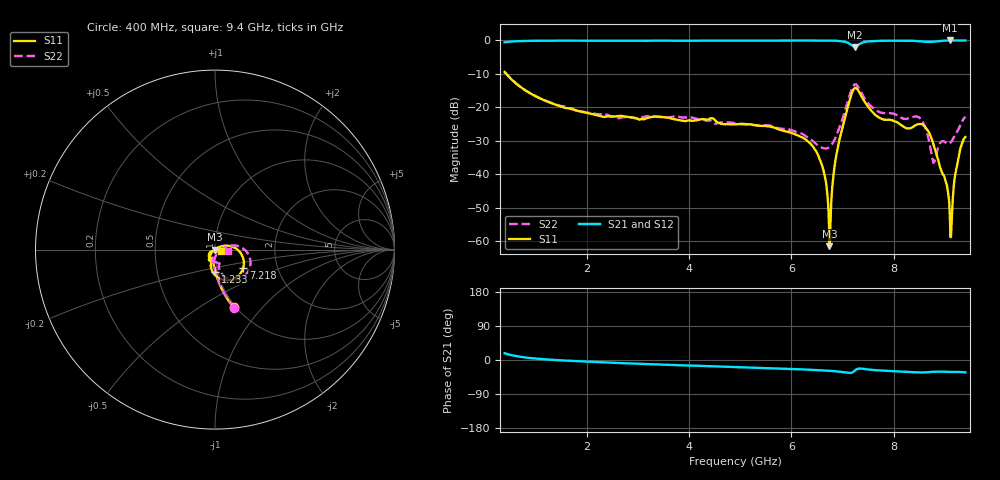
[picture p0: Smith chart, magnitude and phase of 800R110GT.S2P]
!  American Technical Ceramics  Date:  10/25/10
!  One Norden Lane
!  Huntington Station,  NY.  11746-2102
!  Tel:  (631) 622-4700  Fax:  (631) 622-4748
!  Part Number  800R110GT  Mounting Orientation: Vertical
!  Description: Ultra Low ESR Microwave Capacitor
!  Application: Coupling, Bypass, Tuning, DC Block, Filters, Matching
# GHZ S DB R 50
! Freq  |S11|  S11 Ph  |S21|  S21 Ph  |S12|  S12 Ph  |S22|  S22 Ph
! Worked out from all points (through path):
!   801 points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, 400 MHz to 9.4 GHz, reference 50 ohm
!   highest |S21| = 0.00 dB at 9.096 GHz (marker M1); lowest = -1.9 dB at 7.24 GHz (marker M2)
!   group delay of S21, straight-line fit = 12.8 ps
!   lowest |S11| = -61.5 dB at 6.745 GHz (marker M3), VSWR 1.00, Z = 49.9 + j0.0208 ohm
!   |S11| at or under -10 dB: 432.9 MHz to end of sweep
!   |S22| runs from -36.6 to -9.4 dB; largest |S21 - S12| = 0.0024
!   S11 on the Smith chart (normalised r, x): 400 MHz: 0.98, -0.71; 1.233 GHz: 0.97, -0.24; 7.218 GHz: 1.34, -0.28; 9.4 GHz: 1.07, -0.01
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0.4  -9.40 -72.1  -0.53 18.0  -0.53 18.0  -9.37 -71.9
1.233  -18.26 -89.0  -0.07 1.4  -0.07 1.3  -18.20 -88.2
1.908  -21.35 -94.8  -0.05 -3.8  -0.04 -3.8  -21.20 -93.0
3.404  -22.74 -104.4  -0.04 -11.6  -0.03 -11.7  -22.85 -98.3
4.9  -25.07 -116.7  -0.04 -18.6  -0.04 -18.7  -24.72 -100.8
6.408  -31.44 -137.2  -0.01 -26.0  -0.01 -26.0  -29.91 -79.8
6.633  -39.12 -141.8  -0.04 -27.6  -0.04 -27.7  -32.24 -49.6
6.745  -61.50 165.7  -0.05 -28.5  -0.06 -28.6  -31.84 -25.2
6.779  -48.62 47.8  -0.06 -28.9  -0.07 -28.9  -31.29 -17.3
6.824  -40.27 38.4  -0.08 -29.3  -0.09 -29.4  -30.27 -7.2
6.891  -33.33 33.2  -0.12 -30.2  -0.13 -30.3  -28.01 5.2
7.218  -14.57 -32.3  -1.85 -30.6  -1.85 -30.6  -13.43 -21.7
7.24  -14.22 -43.3  -1.91 -28.0  -1.91 -28.1  -13.13 -31.3
7.904  -23.69 -103.8  -0.07 -28.9  -0.07 -29.0  -21.73 -71.3
8.489  -24.99 -112.6  -0.21 -32.8  -0.22 -32.9  -22.95 -85.2
8.658  -26.77 -138.1  -0.42 -32.3  -0.42 -32.4  -28.04 -106.4
8.781  -31.32 -153.3  -0.36 -31.1  -0.37 -31.1  -36.58 -66.5
9.018  -42.25 -126.3  -0.04 -31.4  -0.05 -31.4  -30.55 -31.9
9.096  -52.24 -120.0  0.00 -31.6  -0.01 -31.6  -30.81 -18.4
9.141  -50.67 10.6  -0.01 -31.5  -0.01 -31.6  -29.91 -9.0
9.276  -34.14 16.5  -0.01 -31.6  -0.01 -31.7  -26.18 2.2
9.4  -28.86 -9.1  -0.01 -32.6  -0.01 -32.7  -22.79 -5.8
